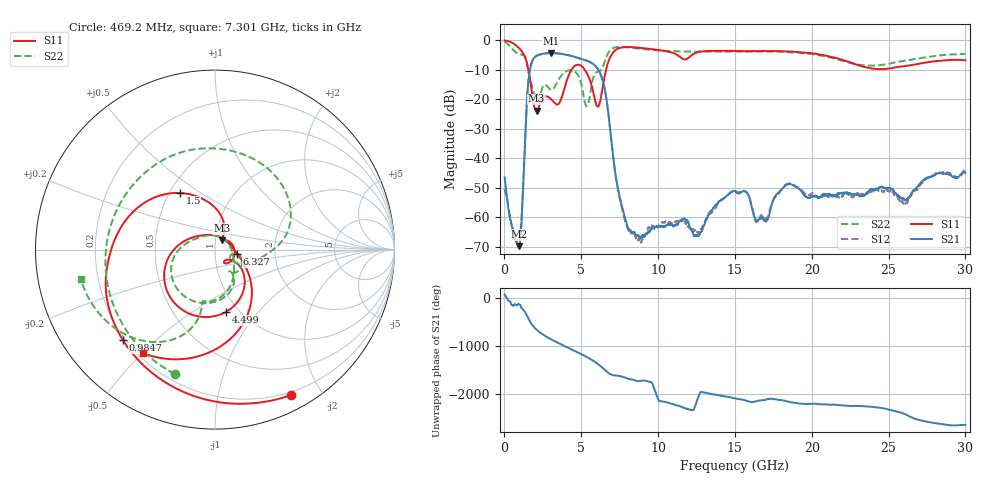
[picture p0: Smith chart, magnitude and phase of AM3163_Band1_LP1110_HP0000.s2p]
!Agilent Technologies,E8364B,MY43040894,A.07.50.67
!Agilent E8364B: A.07.50.67
!Date: Thursday, August 20, 2020 11:30:11
!Correction: S11(Full 2 Port(1,2))
!S21(Full 2 Port(1,2))
!S12(Full 2 Port(1,2))
!S22(Full 2 Port(1,2))
!S2P File: Measurements: S11, S21, S12, S22:
# Hz S  dB  R 50
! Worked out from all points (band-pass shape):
!   3201 points, 10 MHz to 30 GHz, reference 50 ohm
!   highest |S21| = -4.34 dB at 3.028 GHz (marker M1); lowest = -69.7 dB at 956.6 MHz (marker M2)
!   |S21| within 3 dB of the highest: 1.785 GHz to 5.55 GHz (3.765 GHz wide, 103 % of centre)
!   lowest |S11| = -23.8 dB at 2.091 GHz (marker M3), VSWR 1.14, Z = 53.6 + j5.63 ohm
!   |S11| at or under -10 dB: 1.554 GHz to 4.363 GHz (2.808 GHz wide, 94.9 % of centre); 5.227 GHz to 6.612 GHz (1.385 GHz wide, 23.4 % of centre)
!   |S22| runs from -22.3 to -0.4 dB; largest |S21 - S12| = 0.003
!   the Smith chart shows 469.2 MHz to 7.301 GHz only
!   S11 on the Smith chart (normalised r, x): 469.2 MHz: 0.17, -1.64; 984.7 MHz: 0.19, -0.40; 1.5 GHz: 0.56, +0.41; 4.499 GHz: 0.87, -0.69; 6.327 GHz: 1.28, -0.06; 7.301 GHz: 0.22, -0.50
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1e7  -0.08 -8.7  -46.44 64.7  -50.49 26.4  -0.42 -16.9
4.692219e8  -0.78 -62.4  -62.68 -149.1  -62.63 -97.4  -2.75 -107.9
9.565594e8  -2.71 -131.2  -69.74 -140.7  -67.74 114.7  -4.66 147.7
9.84675e8  -2.86 -135.6  -69.25 -143.5  -67.18 -179.0  -4.70 141.3
1.500128e9  -8.60 121.9  -17.51 -39.1  -17.49 -39.3  -9.09 3.7
2.090556e9  -23.83 54.4  -5.29 51.6  -5.29 51.6  -20.37 -29.3
2.615381e9  -19.06 -10.2  -4.49 -70.8  -4.50 -70.8  -15.07 -36.7
3.027744e9  -19.91 -49.5  -4.34 -146.9  -4.35 -146.9  -16.78 -57.3
3.749378e9  -18.99 -32.4  -4.64 96.2  -4.66 96.2  -11.67 -74.9
4.499128e9  -9.06 -80.0  -5.53 -18.6  -5.55 -18.3  -10.32 -132.7
5.014581e9  -8.77 -133.3  -6.36 -98.3  -6.33 -98.2  -15.07 171.9
5.829934e9  -18.81 137.3  -8.30 114.1  -8.32 113.9  -12.02 -77.3
6.326644e9  -17.95 -10.9  -12.49 -6.3  -12.54 -6.2  -9.77 -103.0
7.301319e9  -3.07 -125.0  -47.95 176.5  -48.10 177.2  -2.32 -167.8
8.182275e9  -2.31 173.0  -64.68 101.5  -64.66 111.0  -2.52 141.8
1.000979e10  -3.30 85.7  -62.95 34.3  -63.17 11.7  -3.46 64.9
1.279324e10  -3.83 -2.9  -64.92 -168.2  -63.99 129.9  -3.86 -30.8
1.5005e10  -3.62 -71.6  -51.08 60.6  -51.31 60.3  -3.80 -92.0
2.000958e10  -4.42 163.4  -52.89 -51.6  -51.83 -55.4  -4.70 136.5
2.274617e10  -7.99 60.8  -52.04 -96.8  -52.80 -96.4  -7.97 21.4
2.500479e10  -9.62 -62.3  -50.15 -170.1  -51.10 -165.0  -7.98 -92.5
3e10  -6.81 104.8  -44.82 -131.4  -43.08 -131.6  -4.66 102.5
